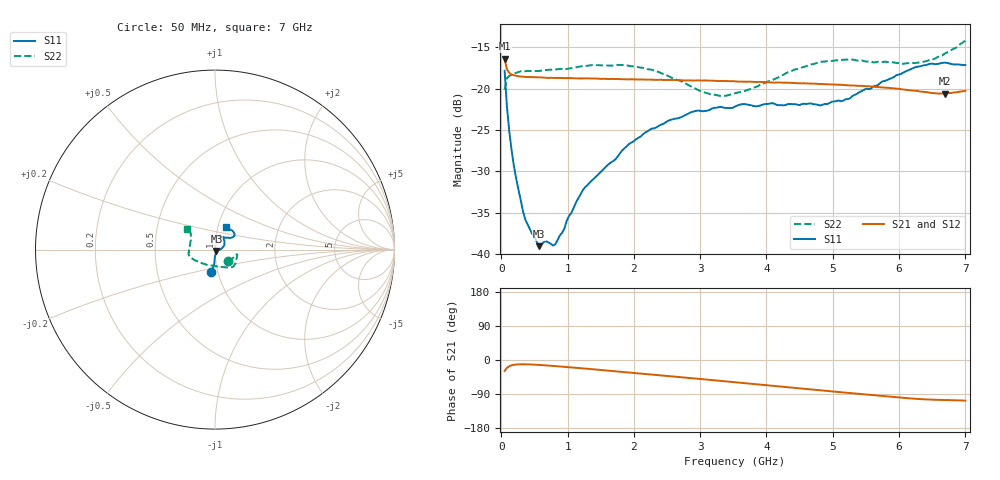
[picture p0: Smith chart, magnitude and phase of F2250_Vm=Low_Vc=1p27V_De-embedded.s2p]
! Integrated Device Technology
! Corporate Headquarters
! 6024 Silver Creek Valley Road
! San Jose, CA 95138  USA
! Phone:  1-408-284-8200
! Toll Free:  1-800-223-1366
! Webpage:  http://www.idt.com/
! Timing and RF Division
! 515 Groton Road, Suite 102
! Westford, MA 01886-6024
! Device:  F2250
! Description: Voltage Variable RF Attenuator
! Frequency:  50.0 -  6000.00 MHz
! Package:  3x3 mm Thin QFN Plastic Package: 16 pin
! Ports:  2 RF, 3 DC
!  Pin  1  = GND
!  Pin  2  = NC
!  Pin  3  = RF1  = Port 1
!  Pin  4  = NC
!  Pin  5  = GND
!  Pin  6  = GND
!  Pin  7  = GND
!  Pin  8  = GND
!  Pin  9  = NC
!  Pin 10  = RF2  = Port 2
!  Pin 11  = NC
!  Pin 12  = GND
!  Pin 13  = GND
!  Pin 14  = VCNTRL
!  Pin 15  = VDD
!  Pin 16  = VMODE
! Vcntrl:  1.270 Volts
! Vmode:  +0.000 Volts
! Vdd:  +3.30  Volts
! Current:  1.192 mA
! Data:  The device was measured on a the F2250 evaluation board which has
!  individual transmission lines to the RF pins.  Data was collected
!  using a calibrated network analyzer.  The evaluation board was
!  de-embedded using a TRL calibration technique.
!  The reference plane is the edge of the package pin.
! Misc:  SN 10
!  Action Tracker AT0258
! Date Measured:  2014-11-26
! Date:  2015-10-15  MJV
! Note:
!  Integrated Device Technology supplies this data as a sample of measured
!  data at the package pin for this product.  Your particular data for this
!  product may vary.
!  Data was taken at 25 degrees C.
!  Integrated Device Technology reserves the right to change this data at anytime.
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# GHz S dB R 50
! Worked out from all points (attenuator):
!   201 points, 50 MHz to 7 GHz, reference 50 ohm
!   highest |S21| = -16.39 dB at 50 MHz (marker M1); lowest = -20.6 dB at 6.687 GHz (marker M2)
!   lowest |S11| = -39.0 dB at 571.2 MHz (marker M3), VSWR 1.02, Z = 50.8 - j0.792 ohm
!   |S11| at or under -10 dB: start of sweep to end of sweep
!   |S22| runs from -20.9 to -14.2 dB; largest |S21 - S12| = 0.00054
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0.05  -17.85 -99.5  -16.39 -29.0  -16.40 -29.0  -20.10 -42.1
0.08475  -22.15 -93.0  -17.66 -20.6  -17.66 -20.6  -18.74 -20.5
0.1195  -25.09 -92.0  -18.09 -16.4  -18.09 -16.4  -18.47 -14.7
0.15425  -27.37 -91.4  -18.29 -14.1  -18.27 -14.0  -18.35 -12.9
0.22375  -30.83 -84.5  -18.45 -11.9  -18.48 -11.9  -18.10 -12.5
0.36275  -35.82 -73.9  -18.58 -11.3  -18.60 -11.3  -17.89 -13.1
0.57125  -39.02 -44.1  -18.63 -13.0  -18.64 -13.0  -17.86 -17.9
0.6755  -38.42 -37.8  -18.69 -14.2  -18.69 -14.3  -17.76 -20.4
0.8145  -38.80 -21.6  -18.71 -16.1  -18.70 -16.1  -17.69 -24.3
1.2315  -32.23 -4.4  -18.77 -22.1  -18.75 -22.1  -17.26 -33.8
1.9265  -26.69 17.3  -18.88 -32.8  -18.86 -32.9  -17.24 -44.9
2.37825  -24.47 28.5  -18.93 -40.0  -18.92 -40.0  -17.99 -53.2
2.86475  -22.84 43.5  -19.02 -47.9  -19.00 -47.9  -19.73 -69.5
3.108  -22.66 50.7  -19.03 -51.9  -19.04 -51.9  -20.56 -83.0
3.35125  -22.29 59.8  -19.07 -55.9  -19.07 -55.9  -20.89 -99.4
3.525  -22.17 62.8  -19.12 -58.7  -19.13 -58.7  -20.56 -111.6
4.7065  -21.88 67.7  -19.40 -78.2  -19.39 -78.2  -17.03 -160.6
5.22775  -21.26 50.7  -19.60 -86.8  -19.59 -86.8  -16.50 -170.0
5.85325  -18.83 35.6  -19.91 -96.9  -19.90 -96.9  -16.82 176.5
6.33975  -17.25 37.8  -20.36 -103.4  -20.34 -103.5  -16.80 159.2
6.68725  -16.86 46.6  -20.60 -105.4  -20.57 -105.5  -15.77 146.4
7  -17.16 62.9  -20.26 -107.3  -20.25 -107.4  -14.18 143.8
